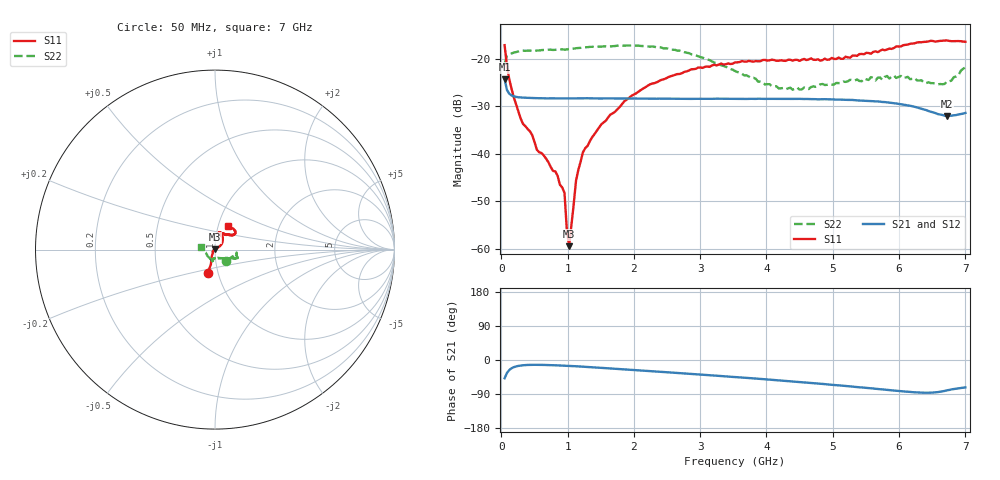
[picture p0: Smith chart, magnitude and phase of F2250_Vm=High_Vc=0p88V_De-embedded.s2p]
! Integrated Device Technology
! Corporate Headquarters
! 6024 Silver Creek Valley Road
! San Jose, CA 95138  USA
! Phone:  1-408-284-8200
! Toll Free:  1-800-223-1366
! Webpage:  http://www.idt.com/
! Timing and RF Division
! 515 Groton Road, Suite 102
! Westford, MA 01886-6024
! Device:  F2250
! Description: Voltage Variable RF Attenuator
! Frequency:  50.0 -  6000.00 MHz
! Package:  3x3 mm Thin QFN Plastic Package: 16 pin
! Ports:  2 RF, 3 DC
!  Pin  1  = GND
!  Pin  2  = NC
!  Pin  3  = RF1  = Port 1
!  Pin  4  = NC
!  Pin  5  = GND
!  Pin  6  = GND
!  Pin  7  = GND
!  Pin  8  = GND
!  Pin  9  = NC
!  Pin 10  = RF2  = Port 2
!  Pin 11  = NC
!  Pin 12  = GND
!  Pin 13  = GND
!  Pin 14  = VCNTRL
!  Pin 15  = VDD
!  Pin 16  = VMODE
! Vcntrl:  0.880 Volts
! Vmode:  +3.300 Volts
! Vdd:  +3.30  Volts
! Current:  1.312 mA
! Data:  The device was measured on a the F2250 evaluation board which has
!  individual transmission lines to the RF pins.  Data was collected
!  using a calibrated network analyzer.  The evaluation board was
!  de-embedded using a TRL calibration technique.
!  The reference plane is the edge of the package pin.
! Misc:  SN 10
!  Action Tracker AT0258
! Date Measured:  2014-11-26
! Date:  2015-10-15  MJV
! Note:
!  Integrated Device Technology supplies this data as a sample of measured
!  data at the package pin for this product.  Your particular data for this
!  product may vary.
!  Data was taken at 25 degrees C.
!  Integrated Device Technology reserves the right to change this data at anytime.
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# GHz S dB R 50
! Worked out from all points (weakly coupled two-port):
!   201 points, 50 MHz to 7 GHz, reference 50 ohm
!   highest |S21| = -24.32 dB at 50 MHz (marker M1); lowest = -32.1 dB at 6.722 GHz (marker M2)
!   lowest |S11| = -59.5 dB at 1.023 GHz (marker M3), VSWR 1.00, Z = 50 + j0.106 ohm
!   |S11| at or under -10 dB: start of sweep to end of sweep
!   |S22| runs from -26.5 to -17.2 dB; largest |S21 - S12| = 0.00016
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0.05  -17.17 -107.1  -24.32 -48.1  -24.31 -48.1  -21.05 -44.0
0.08475  -21.49 -105.6  -26.59 -34.3  -26.57 -34.3  -19.39 -19.6
0.1195  -24.27 -109.6  -27.38 -26.5  -27.39 -26.5  -19.08 -12.9
0.29325  -32.65 -122.2  -28.19 -14.6  -28.16 -14.5  -18.36 -9.0
0.467  -36.11 -140.0  -28.29 -12.7  -28.27 -12.7  -18.36 -8.7
0.5365  -39.19 -147.2  -28.34 -12.7  -28.32 -12.7  -18.30 -9.8
0.8145  -43.75 172.2  -28.38 -14.0  -28.36 -14.0  -18.16 -13.5
0.9535  -48.29 176.6  -28.40 -15.0  -28.39 -15.0  -18.13 -15.5
0.98825  -55.97 172.3  -28.39 -15.3  -28.38 -15.3  -18.06 -15.9
1.023  -59.50 92.7  -28.40 -15.6  -28.39 -15.6  -17.97 -16.0
1.12725  -45.69 34.7  -28.37 -16.5  -28.37 -16.5  -17.81 -17.3
1.2315  -39.73 28.8  -28.36 -17.6  -28.36 -17.6  -17.64 -18.8
1.5095  -33.83 34.5  -28.39 -20.7  -28.39 -20.8  -17.50 -20.3
1.857  -28.97 35.8  -28.41 -24.7  -28.42 -24.7  -17.26 -22.1
2.37825  -24.74 44.4  -28.43 -30.9  -28.44 -30.9  -17.58 -23.9
2.969  -21.89 58.3  -28.47 -37.9  -28.47 -38.0  -19.52 -26.8
3.525  -20.80 70.7  -28.49 -44.9  -28.51 -45.0  -22.61 -41.5
4.18525  -20.45 76.7  -28.48 -53.5  -28.48 -53.5  -26.28 -70.9
4.7065  -20.24 71.4  -28.53 -61.1  -28.52 -61.1  -25.85 -95.4
5.85325  -17.89 39.9  -29.27 -79.4  -29.30 -79.5  -24.20 -102.1
6.722  -16.18 48.9  -32.06 -80.0  -32.06 -80.1  -24.82 -165.1
7  -16.45 62.0  -31.44 -72.2  -31.41 -72.4  -21.86 168.0
